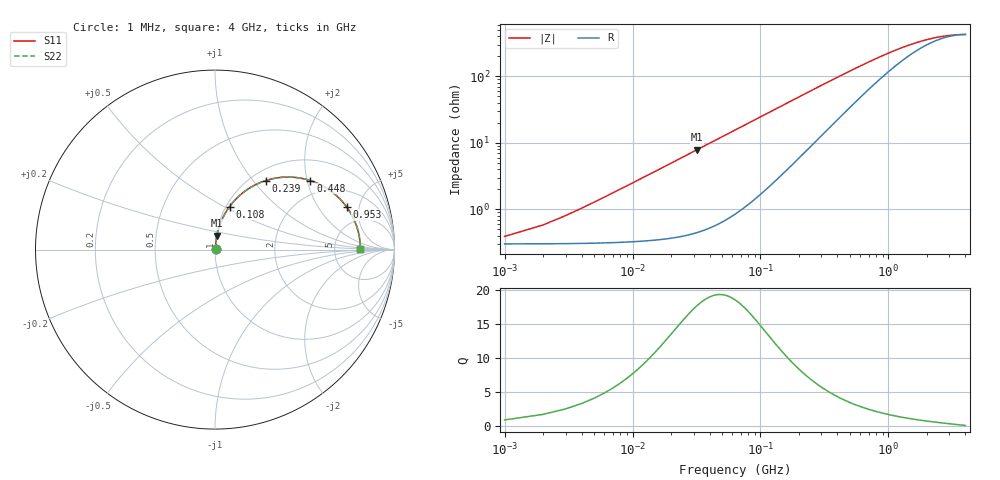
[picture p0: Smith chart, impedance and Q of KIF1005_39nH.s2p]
!version-2
!date-12.2020
!Series
# MHz S RI R 50
!Freq ReS11 ImS11 ReS21 ImS21 ReS12 ImS12 ReS22 ImS22
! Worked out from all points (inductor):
!   4000 points, 1 MHz to 4 GHz, reference 50 ohm
!   read as one part in series: L = 39.1 nH near 21 MHz
!   highest Q = 17.7 at 32 MHz (marker M1), where L = 39.1 nH
!   S11 on the Smith chart (normalised r, x): 1 MHz: 1.01, +0.00; 108 MHz: 1.04, +0.53; 239 MHz: 1.17, +1.16; 448 MHz: 1.55, +2.10; 953 MHz: 3.17, +3.72; 4 GHz: 9.56, +0.10
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1  0.003 0.00246  0.997 -0.00246  0.997 -0.00246  0.003 0.00246
11  0.00399 0.0269  0.996 -0.0269  0.996 -0.0269  0.00399 0.0269
23  0.00696 0.0559  0.993 -0.0559  0.993 -0.0559  0.00696 0.0559
27  0.00839 0.0655  0.9916 -0.0655  0.9916 -0.0655  0.00839 0.0655
32  0.0105 0.0775  0.9895 -0.0775  0.9895 -0.0775  0.0105 0.0775
45  0.0176 0.1081  0.9824 -0.1081  0.9824 -0.1081  0.0176 0.1081
62  0.0303 0.1466  0.9697 -0.1466  0.9697 -0.1466  0.0303 0.1466
83  0.0508 0.1914  0.9492 -0.1914  0.9492 -0.1914  0.0508 0.1914
108  0.081 0.2394  0.919 -0.2394  0.919 -0.2394  0.081 0.2394
135  0.119 0.2839  0.881 -0.2839  0.881 -0.2839  0.119 0.2839
165  0.1651 0.3241  0.8349 -0.3241  0.8349 -0.3241  0.1651 0.3241
239  0.2828 0.3848  0.7172 -0.3848  0.7172 -0.3848  0.2828 0.3848
330  0.4105 0.4041  0.5895 -0.4041  0.5895 -0.4041  0.4105 0.4041
448  0.532 0.3842  0.468 -0.3842  0.468 -0.3842  0.532 0.3842
550  0.6035 0.3529  0.3965 -0.3529  0.3965 -0.3529  0.6035 0.3529
668  0.6598 0.3149  0.3402 -0.3149  0.3402 -0.3149  0.6598 0.3149
953  0.733 0.2382  0.267 -0.2382  0.267 -0.2382  0.733 0.2382
1334  0.7734 0.1695  0.2266 -0.1695  0.2266 -0.1695  0.7734 0.1695
2001  0.7983 0.0989  0.2017 -0.0989  0.2017 -0.0989  0.7983 0.0989
2667  0.8067 0.0562  0.1933 -0.0562  0.1933 -0.0562  0.8067 0.0562
3334  0.8098 0.0258  0.1902 -0.0258  0.1902 -0.0258  0.8098 0.0258
4000  0.8106 0.00173  0.1894 -0.00173  0.1894 -0.00173  0.8106 0.00173
